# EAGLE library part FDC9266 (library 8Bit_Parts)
FDC9266 MFM Disk Controller
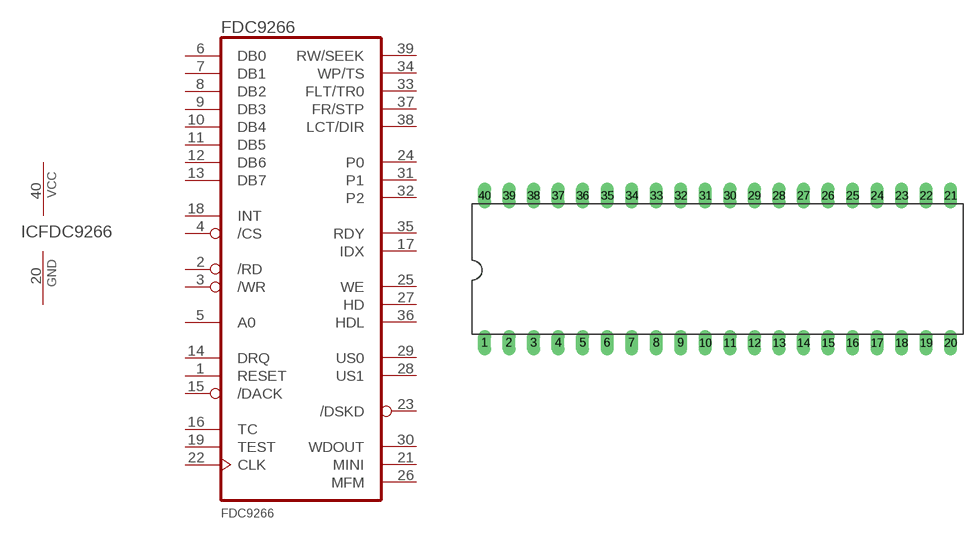
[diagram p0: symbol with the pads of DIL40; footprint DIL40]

Designator prefix IC; gates G$1=FDC9266 FDC9266=PWRN

## FDC9266  [DIL40]
1  G$1:RESET  in
2  G$1:/RD  out
3  G$1:/WR  out
4  G$1:/CS  out
5  G$1:A0  hiz
6  G$1:DB0
7  G$1:DB1
8  G$1:DB2
9  G$1:DB3
10  G$1:DB4
11  G$1:DB5
12  G$1:DB6
13  G$1:DB7
14  G$1:DRQ  in
15  G$1:/DACK  out
16  G$1:TC  in
17  G$1:IDX  in
18  G$1:INT  in
19  G$1:TEST  nc
20  FDC9266:GND  pwr
21  G$1:MINI  in
22  G$1:CLK  in
23  G$1:/DSKD  in
24  G$1:P0  hiz
25  G$1:WE  out
26  G$1:MFM  out
27  G$1:HD  out
28  G$1:US1  out
29  G$1:US0  out
30  G$1:WDOUT  out
31  G$1:P1  hiz
32  G$1:P2  hiz
33  G$1:FLT/TR0  in
34  G$1:WP/TS  in
35  G$1:RDY  in
36  G$1:HDL  out
37  G$1:FR/STP  hiz
38  G$1:LCT/DIR  hiz
39  G$1:RW/SEEK  hiz
40  FDC9266:VCC  pwr

## Footprint DIL40 (pad centres in mm)
Dual In Line Package
drill 0.813 long: 1 -24.13,-7.62; 2 -21.59,-7.62; 3 -19.05,-7.62; 4 -16.51,-7.62; 5 -13.97,-7.62; 6 -11.43,-7.62; 7 -8.89,-7.62; 8 -6.35,-7.62; 9 -3.81,-7.62; 10 -1.27,-7.62; 11 1.27,-7.62; 12 3.81,-7.62; 13 6.35,-7.62; 14 8.89,-7.62; 15 11.43,-7.62; 16 13.97,-7.62; 17 16.51,-7.62; 18 19.05,-7.62; 19 21.59,-7.62; 20 24.13,-7.62; 21 24.13,7.62; 22 21.59,7.62; 23 19.05,7.62; 24 16.51,7.62; 25 13.97,7.62; 26 11.43,7.62; 27 8.89,7.62; 28 6.35,7.62; 29 3.81,7.62; 30 1.27,7.62; 31 -1.27,7.62; 32 -3.81,7.62; 33 -6.35,7.62; 34 -8.89,7.62; 35 -11.43,7.62; 36 -13.97,7.62; 37 -16.51,7.62; 38 -19.05,7.62; 39 -21.59,7.62; 40 -24.13,7.62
